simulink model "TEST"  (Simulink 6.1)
settings: Solver=ode45  StartTime=0.0  StopTime=4  RelTol=1e-3
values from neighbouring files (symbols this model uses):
  a = axes( 'Parent',  centerPanel,   'Projection', 'perspective',   'CameraPosition',[-9.75 -7.705 11.42],   'CameraUpVector',[0.4677 0.3787 0.7986],   'Color',[1 1 1],   'NextPlot', 'replacechildren',   'XColor',kColor(1,:),   'YColor',kColor(2,:),   'ZColor',kColor(3,:),   'Position',[0.1 0.1 0.8 0.8],   'Visible', 'off')    [SAUAnalizeProject.m]    (also in TESTm.m = 0.001; slpriv1m.m = 0.001; red1m.m = 0.001)
  ak0 = 1    [TESTm.m]    (also in slpriv1m.m)
  ak1 = 0.5    [TESTm.m]    (also in slpriv1m.m)
  ap0 = 1    [TESTm.m]    (also in slpriv1m.m)
  ap1 = 0.001    [TESTm.m]    (also in slpriv1m.m)
  bk0 = 0    [TESTm.m]    (also in slpriv1m.m)
  bk1 = 0.5    [TESTm.m]    (also in slpriv1m.m)
  bp0 = 1    [TESTm.m]    (also in slpriv1m.m)
  bp1 = 0.001    [TESTm.m]    (also in slpriv1m.m)
  c = 2000000    [TESTm.m]    (also in slpriv1m.m; red1m.m)
  F1 = 0    [TESTm.m]    (also in main5.m = peaks(35); main7.m = zeros(A1n,A2n); slpriv1m.m; red1m.m)
  F2 = 0    [TESTm.m]    (also in main5.m = membrane; main7.m = zeros(A1n,A2n); slpriv1m.m; red1m.m)
  G = 0    [TESTm.m]    (also in slpriv1m.m; red1m.m)
  G1 = 0    [TESTm.m]    (also in slpriv1m.m; red1m.m)
  G2 = 0    [TESTm.m]    (also in slpriv1m.m; red1m.m)
  i = find( isoLevel == src )    [SAUAnalizeProject.m]    (also in TESTm.m = 100; slpriv1m.m = 100; red1m.m = 100)
  J = 0.04    [TESTm.m]    (also in slpriv1m.m)
  Jn = 200    [TESTm.m]    (also in slpriv1m.m; red1m.m)
  k1 = 1/R    (= 2)    [TESTm.m]    (also in myparam.m; slpriv1m.m)
  Kc = 0.0015    [TESTm.m]    (also in slpriv1m.m)
  Ki = 0.0003    [TESTm.m]    (also in slpriv1m.m)
  kip = 0    [TESTm.m]    (also in slpriv1m.m)
  Kk = 22500    [TESTm.m]    (also in slpriv1m.m)
  km = 0.36    [TESTm.m]    (also in myparam.m; slpriv1m.m)
  kp = 1    [TESTm.m]    (also in main9.m = 0.5; myfunpole.m = K1; slpriv1m.m)
  kpd = 0    [TESTm.m]    (also in slpriv1m.m)
  kv = 0.45    [TESTm.m]    (also in myparam.m; slpriv1m.m)
  T = L/R    (= 0.02)    [TESTm.m]    (also in myparam.m; slpriv1m.m)
libraries: slctrlobsolete x2

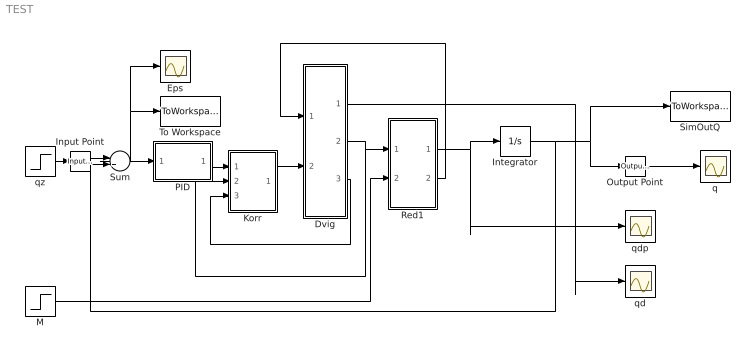
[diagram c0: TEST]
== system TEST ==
  Dvig : Subsystem  AncestorBlock=simulink3/Signals & Systems/SubSystem
  Eps : Scope
  Input Point : slctrlobsolete/Input Point
  Integrator : Integrator
  Korr : Subsystem
  M : Step  Time=0  After=0  SampleTime=0
  Output Point : slctrlobsolete/Output Point
  PID : Subsystem
  Red1 : Subsystem
  SimOutQ : ToWorkspace  VariableName=simoutq  SampleTime=-1  SaveFormat=Structure With Time
  Sum : Sum  Inputs=|+-
  To Workspace : ToWorkspace  VariableName=simouteps  SampleTime=-1  SaveFormat=Structure
  q : Scope
  qd : Scope
  qdp : Scope
  qz : Step  Time=0  SampleTime=0
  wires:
  Sum/1 -> PID/1(eps), Eps/1, To Workspace/1
  PID/1(ueps) -> Korr/1(u_eps)
  Red1/2(M2M) -> Dvig/1(Mv)
  Korr/1(u_d) -> Dvig/2(u)
  Dvig/2(qd') -> Red1/1(q1p), Korr/2(qdp)
  Dvig/3(ia) -> Korr/3(ia)
  M/1 -> Red1/2(-M2)
  Red1/1(q2p) -> Integrator/1, qdp/1
  Integrator/1 -> Sum/2, Output Point/1, SimOutQ/1
  Dvig/1(qd) -> qd/1
  qz/1 -> Input Point/1
  Input Point/1 -> Sum/1
  Output Point/1 -> q/1

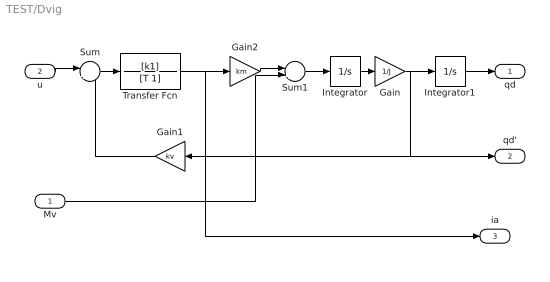
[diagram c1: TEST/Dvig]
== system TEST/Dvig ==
  Mv : Inport  Port=1  LatchInput=off
  u : Inport  Port=2  LatchInput=off
  Gain : Gain  Gain=1/J
  Gain1 : Gain  Orientation=left  Gain=kv
  Gain2 : Gain  Gain=km
  Integrator : Integrator
  Integrator1 : Integrator
  Sum : Sum  Inputs=|+-
  Sum1 : Sum  Inputs=|++
  Transfer Fcn : TransferFcn  Numerator=[k1]  Denominator=[T 1]
  qd : Outport
  qd' : Outport  Port=2
  ia : Outport  Port=3
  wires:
  u/1 -> Sum/1
  Gain1/1 -> Sum/2
  Sum/1 -> Transfer Fcn/1
  Transfer Fcn/1 -> Gain2/1, ia/1
  Gain2/1 -> Sum1/1
  Mv/1 -> Sum1/2
  Sum1/1 -> Integrator/1
  Integrator/1 -> Gain/1
  Gain/1 -> Integrator1/1, Gain1/1, qd'/1
  Integrator1/1 -> qd/1

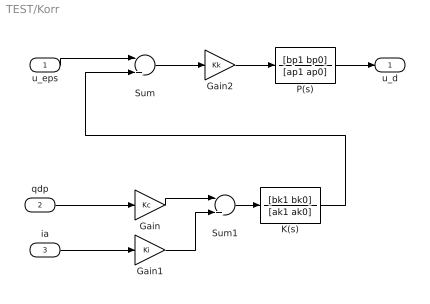
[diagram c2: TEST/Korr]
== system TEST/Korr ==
  u_eps : Inport  Port=1  LatchInput=off
  qdp : Inport  Port=2  LatchInput=off
  ia : Inport  Port=3  LatchInput=off
  Gain : Gain  Gain=Kc
  Gain1 : Gain  Gain=Ki
  Gain2 : Gain  Gain=Kk
  K(s) : TransferFcn  Numerator=[bk1 bk0]  Denominator=[ak1 ak0]
  P(s) : TransferFcn  Numerator=[bp1 bp0]  Denominator=[ap1 ap0]
  Sum : Sum  Inputs=|+-
  Sum1 : Sum  Inputs=|++
  u_d : Outport
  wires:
  u_eps/1 -> Sum/1
  qdp/1 -> Gain/1
  ia/1 -> Gain1/1
  Sum/1 -> Gain2/1
  Gain/1 -> Sum1/1
  Gain1/1 -> Sum1/2
  Gain2/1 -> P(s)/1
  P(s)/1 -> u_d/1
  Sum1/1 -> K(s)/1
  K(s)/1 -> Sum/2

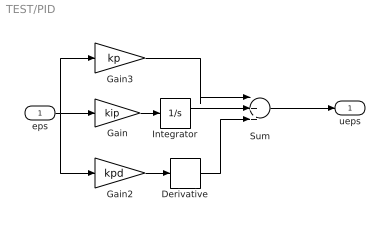
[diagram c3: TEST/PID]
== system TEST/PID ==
  eps : Inport  Port=1  LatchInput=off
  Derivative : Derivative
  Gain : Gain  Gain=kip
  Gain2 : Gain  Gain=kpd
  Gain3 : Gain  Gain=kp
  Integrator : Integrator
  Sum : Sum  Inputs=|+++
  ueps : Outport
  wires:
  Sum/1 -> ueps/1
  Gain/1 -> Integrator/1
  eps/1 -> Gain/1, Gain2/1, Gain3/1
  Integrator/1 -> Sum/2
  Gain2/1 -> Derivative/1
  Derivative/1 -> Sum/3
  Gain3/1 -> Sum/1

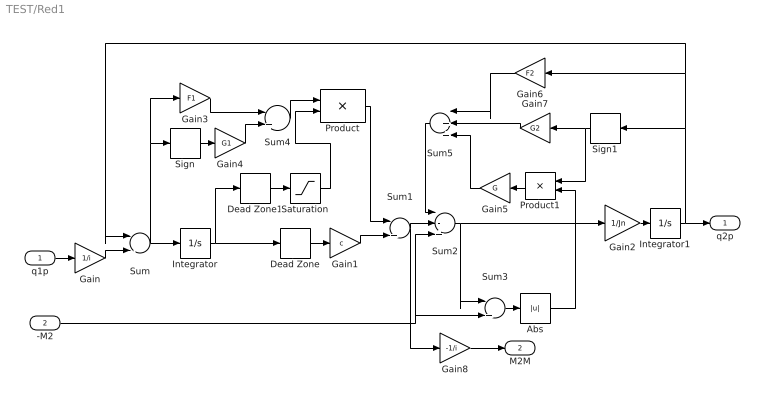
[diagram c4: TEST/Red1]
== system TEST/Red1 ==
  q1p : Inport  Port=1  LatchInput=off
  -M2 : Inport  Port=2  LatchInput=off
  Abs : Abs
  Dead Zone : DeadZone  LowerValue=-a  UpperValue=a
  Dead Zone1 : DeadZone  LowerValue=-a  UpperValue=a
  Gain : Gain  Gain=1/i
  Gain1 : Gain  Gain=c
  Gain2 : Gain  Gain=1/Jn
  Gain3 : Gain  Gain=F1
  Gain4 : Gain  Gain=G1
  Gain5 : Gain  Orientation=left  Gain=G
  Gain6 : Gain  Orientation=left  Gain=F2
  Gain7 : Gain  Orientation=left  Gain=G2
  Gain8 : Gain  Gain=-1/i
  Integrator : Integrator
  Integrator1 : Integrator
  Product : Product
  Product1 : Product  Orientation=left
  Saturation : Saturate  UpperLimit=a  LowerLimit=-a
  Sign : Signum
  Sign1 : Signum  Orientation=left
  Sum : Sum  Inputs=|-+
  Sum1 : Sum  Inputs=|++
  Sum2 : Sum  Inputs=|-++
  Sum3 : Sum  Inputs=|++
  Sum4 : Sum  Inputs=|++
  Sum5 : Sum  Orientation=left  Inputs=|+++
  q2p : Outport
  M2M : Outport  Port=2
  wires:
  q1p/1 -> Gain/1
  Gain/1 -> Sum/2
  Sum/1 -> Integrator/1, Gain3/1, Sign/1
  Integrator/1 -> Dead Zone/1, Dead Zone1/1
  Dead Zone/1 -> Gain1/1
  Gain1/1 -> Sum1/2
  Sum1/1 -> Sum2/2, Gain8/1
  Sum2/1 -> Gain2/1, Sum3/1
  Gain2/1 -> Integrator1/1
  Integrator1/1 -> q2p/1, Sign1/1, Gain6/1, Sum/1
  -M2/1 -> Sum3/2, Sum2/3
  Sum3/1 -> Abs/1
  Gain3/1 -> Sum4/1
  Gain4/1 -> Sum4/2
  Sign/1 -> Gain4/1
  Sum4/1 -> Product/1
  Product/1 -> Sum1/1
  Sum5/1 -> Sum2/1
  Product1/1 -> Gain5/1
  Gain5/1 -> Sum5/3
  Abs/1 -> Product1/2
  Gain6/1 -> Sum5/1
  Gain7/1 -> Sum5/2
  Sign1/1 -> Gain7/1, Product1/1
  Gain8/1 -> M2M/1
  Dead Zone1/1 -> Saturation/1
  Saturation/1 -> Product/2
